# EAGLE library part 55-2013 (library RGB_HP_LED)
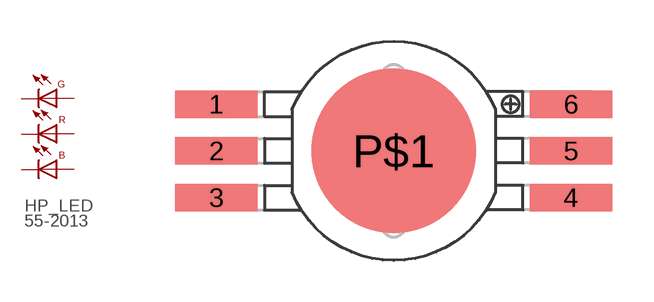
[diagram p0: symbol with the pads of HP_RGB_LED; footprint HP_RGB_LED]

Designator prefix HP_LED

## 55-2013  [HP_RGB_LED]
1  GC  pas
2  RC  pas
3  BC  pas
4  BA  pas
5  RA  pas
6  GA  pas

## Footprint HP_RGB_LED (pad centres in mm)
smd 3 x 1: 1 -6.45,1.7; 2 -6.45,0; 3 -6.45,-1.7; 4 6.45,-1.7; 5 6.45,0; 6 6.45,1.7
smd 6 x 6: P$1 0,0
